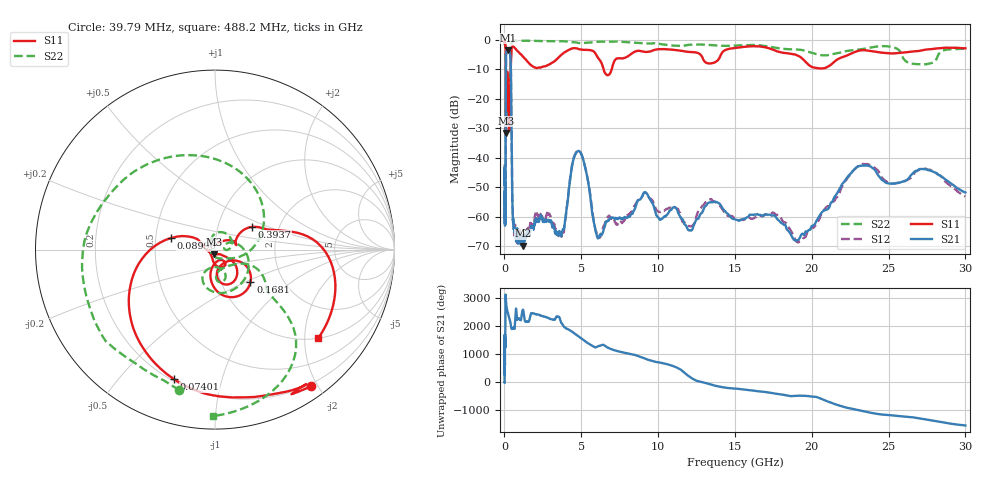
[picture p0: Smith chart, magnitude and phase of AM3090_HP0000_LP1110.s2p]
! Date/Time: Thu, Feb 28, 2019 1:53 PM
! Network Analyzer: Agilent Technologies E8364B Rev: A.07.50.67
! Sweep from 0.010 to 30.000 GHz, 1601 Points, Sweep Type: LOG
! Power Supply: 5.023 V, 0.002 A
# Hz S DB R 50
!freq MagS11 AngS11 MagS21 AngS21 MagS12 AngS12 MagS22 AngS22
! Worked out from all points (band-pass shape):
!   1601 points, 10 MHz to 30 GHz, reference 50 ohm
!   highest |S21| = -3.41 dB at 253.4 MHz (marker M1); lowest = -69.8 dB at 1.238 GHz (marker M2)
!   |S21| within 3 dB of the highest: 100.6 MHz to 396.4 MHz (295.8 MHz wide, 119 % of centre)
!   lowest |S11| = -31.6 dB at 97.94 MHz (marker M3), VSWR 1.05, Z = 49.4 - j2.54 ohm
!   |S11| at or under -10 dB: 88.94 MHz to 408.9 MHz (319.9 MHz wide, 129 % of centre); 6.455 GHz to 6.979 GHz (523.6 MHz wide, 7.8 % of centre)
!   |S22| runs from -32.7 to -0.2 dB; largest |S21 - S12| = 0.012
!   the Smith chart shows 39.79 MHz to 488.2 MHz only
!   S11 on the Smith chart (normalised r, x): 39.79 MHz: 0.17, -1.91; 74.01 MHz: 0.21, -0.71; 89.96 MHz: 0.60, +0.08; 168.1 MHz: 1.37, -0.54; 393.7 MHz: 1.46, +0.39; 488.2 MHz: 1.00, -2.33
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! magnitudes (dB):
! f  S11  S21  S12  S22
! 10 MHz  -0.3  -49.2  -42.3  -0.7
! 38.04 MHz  -0.5  -62.3  -60.4  -1.7
! 39.79 MHz  -0.6  -61.7  -59.2  -1.9
! 74.01 MHz  -2.4  -46.1  -47.6  -4.3
! 89.96 MHz  -11.9  -14.2  -14.3  -12.8
! 97.94 MHz  -31.6  -7.2  -7.2  -32.3
! 144.7 MHz  -18.8  -3.6  -3.6  -24.1
! 168.1 MHz  -11.4  -3.5  -3.5  -14.5
! 253.4 MHz  -22.6  -3.4  -3.4  -17.4
! 312.7 MHz  -31.0  -3.8  -3.8  -16.2
! 393.7 MHz  -12.3  -6.2  -6.2  -10.3
! 488.2 MHz  -2.4  -44.7  -44.5  -0.6
! 550.5 MHz  -2.3  -60.6  -61.2  -0.4
! 1.238 GHz  -5.9  -69.8  -68.1  -0.3
! 2.084 GHz  -9.5  -61.7  -58.8  -0.3
! 3.723 GHz  -5.0  -66.3  -66.8  -0.4
! 4.805 GHz  -3.1  -37.7  -37.6  -1.0
! 6.08 GHz  -6.0  -67.4  -67.2  -0.7
! 7.926 GHz  -5.9  -60.4  -59.7  -0.8
! 19.12 GHz  -5.4  -68.0  -68.8  -3.3
! 23.24 GHz  -3.5  -42.7  -42.2  -3.2
! 30 GHz  -2.9  -51.8  -53.2  -3.0
